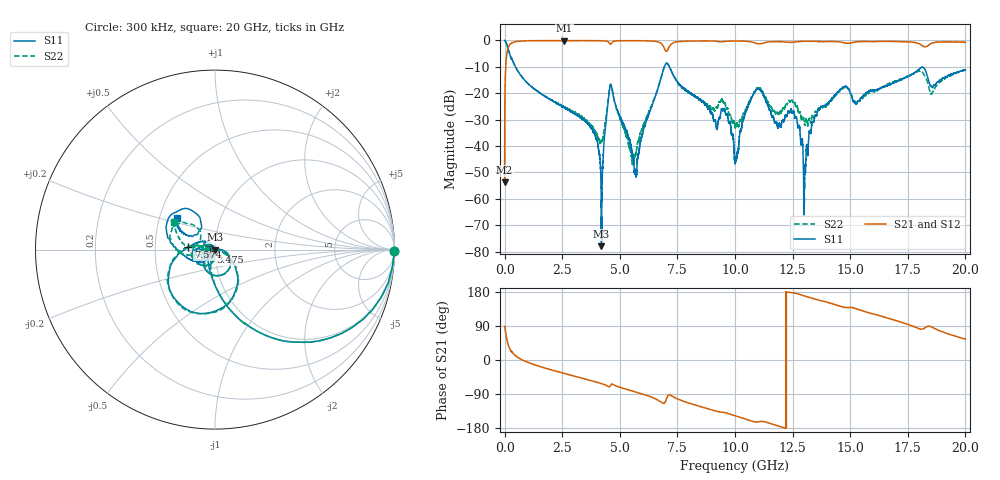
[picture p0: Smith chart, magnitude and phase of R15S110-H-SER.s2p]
!{R15S110}
!Johanson Technology Inc.
!www.johansontechnology.com
!Test Board Conditions:
!Substrate Type  RO4350B
!Substrate Thickness  20 mil
!Substrate Dk  3.66
!TL Type: GCPW
!TL Trace Width  34 mil
!TL Gap  10 mil
!Electrode orientation  Horizontal
!DUT TOPOLOGY	SERIES
!Mounting Pad LxW  26x52 mil
! Created Sat Feb  6 14:07:05 2021
# hz S ma R 50
! 2 Port Network Data from SP1.SP block
! freq  magS11  angS11  magS21  angS21  magS12  angS12  magS22  angS22
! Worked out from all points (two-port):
!   20001 points, 300 kHz to 20 GHz, reference 50 ohm
!   highest |S21| = -0.05 dB at 2.586 GHz (marker M1); lowest = -53.7 dB at 300 kHz (marker M2)
!   |S21| within 3 dB of the highest: 146.3 MHz to 6.938 GHz (6.792 GHz wide, 192 % of centre); 7.11 GHz to end of sweep
!   lowest |S11| = -77.9 dB at 4.205 GHz (marker M3), VSWR 1.00, Z = 50 - j0.0111 ohm
!   |S11| at or under -10 dB: 473.1 MHz to 6.933 GHz (6.46 GHz wide, 174 % of centre); 7.156 GHz to end of sweep
!   |S22| runs from -47.0 to 0.0 dB; largest |S21 - S12| = 0.014
!   S11 on the Smith chart (normalised r, x): 300 kHz: open; 3.475 GHz: 0.95, -0.03; 7.574 GHz: 0.74, +0.02; 20 GHz: 0.61, +0.24
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300000  1 -0.4  0.002058 88.5  0.001994 87.8  0.9974 -0.3
1.053e8  0.8087 -37.6  0.5831 52.3  0.5845 52.2  0.8101 -37.5
2.323e8  0.5309 -61.2  0.8399 28.4  0.8411 28.3  0.5323 -61.2
2.5863e9  0.05352 -133.3  0.9945 -35.4  0.9928 -35.4  0.05585 -112.9
3.3343e9  0.03414 -149.3  0.9924 -47.6  0.9915 -47.6  0.03741 -118.2
3.4753e9  0.03006 -151.8  0.9925 -49.9  0.9922 -49.9  0.033 -118.6
4.2053e9  0.0001273 -61.1  0.987 -62.4  0.9874 -62.4  0.01271 -57.5
4.6013e9  0.1465 -78.0  0.8456 -66.6  0.8463 -66.5  0.1488 -76.3
5.6823e9  0.003312 -91.7  0.9882 -84.2  0.9895 -84.3  0.006955 -32.7
6.6673e9  0.1284 -36.5  0.9384 -106.3  0.9385 -106.3  0.1302 -36.2
7.0353e9  0.3697 -111.6  0.6217 -100.9  0.6213 -100.8  0.374 -112.0
7.5743e9  0.1487 174.6  0.9545 -104.5  0.9554 -104.6  0.1457 175.0
9.5813e9  0.04299 151.4  0.9609 -139.2  0.962 -139.3  0.0607 179.3
1.00003e10  0.004765 138.2  0.9763 -147.0  0.9774 -147.1  0.02375 -152.0
1.09843e10  0.1209 -143.5  0.8675 -163.5  0.8695 -163.4  0.1281 -144.1
1.18073e10  0.02707 173.3  0.95 -172.8  0.9509 -172.8  0.04342 171.4
1.25943e10  0.03638 146.1  0.9351 176.5  0.935 176.4  0.06586 152.1
1.30513e10  0.003528 154.6  0.9648 168.4  0.9659 168.4  0.02761 155.2
1.33343e10  0.02572 -109.9  0.9651 163.3  0.9663 163.2  0.03434 -167.1
1.47263e10  0.1325 -153.4  0.9085 139.1  0.9118 139.2  0.1302 -161.9
1.66673e10  0.1457 -157.0  0.9621 109.8  0.9521 109.6  0.1496 -168.1
2e10  0.2783 140.3  0.9251 54.9  0.9171 54.4  0.2739 145.5
